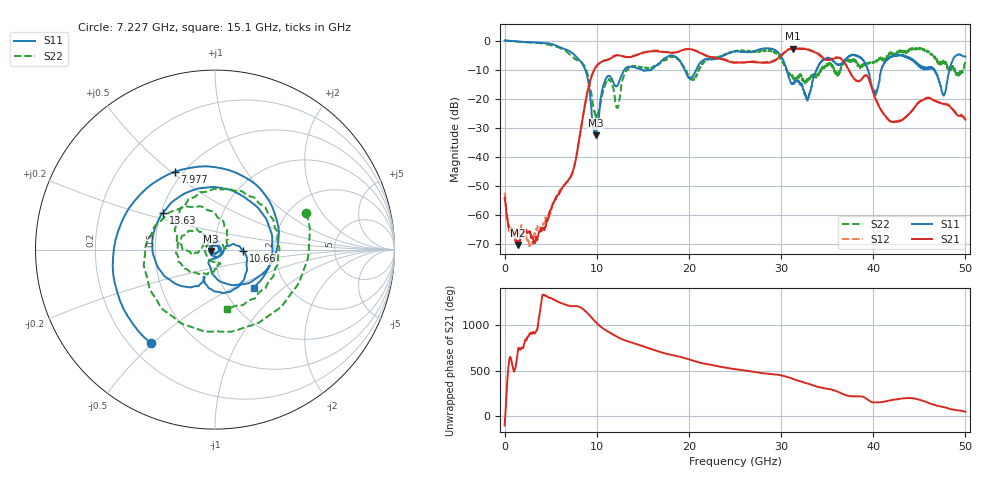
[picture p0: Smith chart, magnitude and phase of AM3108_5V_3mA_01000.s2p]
# Hz S DB R 50.0
!freq dBS11 angS11 dBS21 angS21 dBS12 angS12 dBS22 angS22
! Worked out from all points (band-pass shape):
!   1601 points, 10 MHz to 50 GHz, reference 50 ohm
!   highest |S21| = -2.84 dB at 31.28 GHz (marker M1); lowest = -70.3 dB at 1.416 GHz (marker M2)
!   |S21| within 3 dB of the highest: 11.66 GHz to 22.66 GHz (11.01 GHz wide, 64.1 % of centre); 29.79 GHz to 34.47 GHz (4.68 GHz wide, 14.6 % of centre)
!   lowest |S11| = -32.6 dB at 9.883 GHz (marker M3), VSWR 1.05, Z = 47.9 - j0.802 ohm
!   |S11| at or under -10 dB: 8.751 GHz to 13.01 GHz (4.259 GHz wide, 39.1 % of centre); 30.61 GHz to 33.84 GHz (3.234 GHz wide, 10 % of centre); 46.63 GHz to 48.28 GHz (1.651 GHz wide, 3.48 % of centre)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
!   |S22| runs from -26.8 to 0.0 dB; largest |S21 - S12| = 0.022
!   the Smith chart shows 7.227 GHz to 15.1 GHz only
!   S11 on the Smith chart (normalised r, x): 7.227 GHz: 0.28, -0.49; 7.977 GHz: 0.45, +0.51; 10.66 GHz: 1.37, -0.02; 13.63 GHz: 0.51, +0.24; 15.1 GHz: 1.38, -0.64
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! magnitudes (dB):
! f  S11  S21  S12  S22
! 10 MHz  0.0  -54.1  -52.3  0.0
! 1.416 GHz  -0.3  -70.3  -66.2  -0.4
! 2.916 GHz  -0.6  -67.0  -70.3  -0.7
! 7.227 GHz  -4.0  -46.4  -46.7  -5.2
! 7.977 GHz  -6.2  -36.5  -36.4  -6.8
! 8.352 GHz  -7.5  -29.1  -28.9  -7.4
! 9.883 GHz  -32.6  -9.2  -9.2  -25.6
! 10.66 GHz  -16.1  -7.1  -7.0  -18.1
! 12.26 GHz  -15.4  -5.1  -5.0  -23.2
! 13.63 GHz  -9.0  -5.7  -5.6  -9.2
! 15.1 GHz  -10.4  -4.1  -4.1  -9.4
! 16.69 GHz  -8.1  -3.7  -3.5  -8.3
! 20.41 GHz  -12.2  -3.2  -3.1  -13.6
! 25 GHz  -3.7  -7.6  -7.5  -3.8
! 29.38 GHz  -3.3  -6.8  -6.6  -4.1
! 31.28 GHz  -15.0  -2.8  -2.7  -13.1
! 33.35 GHz  -15.6  -3.7  -3.4  -12.7
! 37.91 GHz  -4.9  -13.1  -13.1  -6.4
! 40.22 GHz  -18.8  -19.8  -19.5  -7.6
! 41.69 GHz  -6.1  -27.3  -27.3  -5.2
! 47.66 GHz  -18.9  -21.8  -21.7  -7.7
! 50 GHz  -5.5  -27.2  -26.7  -6.9
